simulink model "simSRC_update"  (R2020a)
settings: Solver=ode15s  StartTime=0.0  StopTime=tsim  FixedStep=tdelay/2  RelTol=1e-3
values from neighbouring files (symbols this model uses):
  d0 = 0    [runSRC.m]    (also in Main.m = [Fh, Tcin, Thin]; Main_OL.m = [Fh, Tcin, Thin]; runTestCalcBlk.m = [Fh, Tcin, Thin]; runTransf.m = [Fh, Tcin, Thin,U0])
  df = 0    [runSRC.m]
  h0 = x0    [runSRC.m]
  hf = h0    [runSRC.m]
  hmax = [2.3; 2.8; 3.2]    [runSRC.m]    (also in TuneSRC.m)
  nd = length(d0)    [runSRC.m]    (also in Main.m = size(d0,2); Main_OL.m = size(d0,2); runTestCalcBlk.m = size(d0,2); runTransf.m = size(d0,2))
  np = length(param)    [runSRC.m]    (also in runH2Psim.m; Main.m = size(p,2); Main_OL.m = size(p,2); runTestCalcBlk.m = size(p,2))
  nu = length(z0)    [runSRC.m]    (also in runH2Psim.m = length(u0); Main.m = 1; Main_OL.m = 1; runTestCalcBlk.m = 1)
  nx = length(x0)    [runSRC.m]    (also in H2P_Turbine_driven.m = param(end); runTD.m; H2P_Boiler_driven.m = param(end); runBD.m)
  param = [A; Cv; DP; rho; N]    [runSRC.m]    (also in TuneSRC.m = [vmin; vmax; umin; umax; n; price;opening]; runTD.m = [Tref;TrefB;dHvap;cpg;cpW;cpSt;R;Mwt;     T0;TG0;ME;pC;     ; runBD.m = [Tref;TrefB;dHvap;cpg;cpW;cpSt;R;Mwt;          T0;TG0;ME;pC;; runFP.m = [Tref;TrefB;dHvap;cpg;cpW;cpSt;R;Mwt;          T0;TG0;ME;pC;)
  pSR1 = [u01, alpha1, MV]    [runSRC.m]
  pSR2 = [u02, alpha2, MV]    [runSRC.m]
  pSR3 = [u03, alpha3, MV]    [runSRC.m]
  td = 0    [runSRC.m]
  tdelay = 1    [runSRC.m]
  th = ones(6,1)    [runSRC.m]
  v0 = v(end,:)    [runTD.m]    (also in runBD.m; runFP.m; runFPV2.m; runVPC.m)
  x0 = pr/100*hmax    [runSRC.m]    (also in TuneSRC.m = [hH; hH; hH].*hmax; runTD.m = [TE0;TD0;TSh0;MD0; MSh0;w0;TA0;0;0;0;0;0;0;0;0;0]; runBD.m = [TE0;TD0;TSh0;MD0; MSh0;w0;TA0;0;0;0;0;0;0;0;0;0]; runFP.m = [TE0;TD0;TSh0;MD0; MSh0;w0;TA0;0;0;0;0;0;0;0])
  z0 = [0.6; 0.7; 0.8; 1]    [runSRC.m]    (also in TuneSRC.m; runTD.m = [TGE0;TGD;TGSh;pT; Pm0;mG;zV]; runBD.m = [TGE0;TGD;TGSh;pT; Pm0;mG;zV]; runFP.m = [TGE0;TGD;TGSh;pT; Pm0;mG;zV])
  zOP = zOP0-[0.7;0;0;0]    [runSRC.m]
undefined symbols (not defined in the file or in its folder): KcSRC, KISRC, TanksODE, tzOP

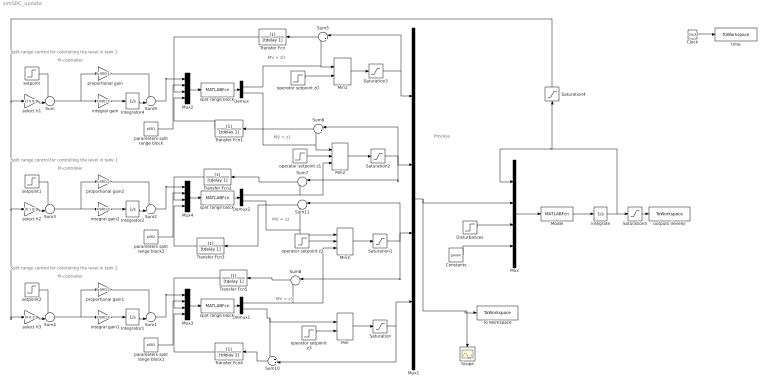
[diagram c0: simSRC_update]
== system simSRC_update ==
  note: MV = z3
  note: MV = z2
  note: MV = z1
  note: MV = z0
  note: Process
  note: Split range control for controlling the level in tank 1
  note: PI-controller
  note: PI-controller
  note: Split range control for controlling the level in tank 2
  note: PI-controller
  note: Split range control for controlling the level in tank 1
  Clock : Clock
  Constants : Constant  Value=param
  Demux : Demux  Outputs=2
  Demux1 : Demux  Outputs=2
  Demux2 : Demux  Outputs=2
  Disturbances : Step  Time=td  Before=d0  After=df  SampleTime=0
  Integrator1 : Integrator  InitialCondition=v0(3)
  Integrator2 : Integrator  InitialCondition=v0(2)
  Integrator4 : Integrator  InitialCondition=v0(1)
  Min : MinMax  Inputs=2
  Min1 : MinMax  Inputs=2
  Min2 : MinMax  Inputs=3
  Min3 : MinMax  Inputs=3
  Model : MATLABFcn  MATLABFcn=TanksODE(u(1:nx),u(nx+1:nx+nu),u(nx+nu+1:nx+nu+nd),u(nx+nu+nd+1:nx+nu+nd+np))  OutputDimensions=nx
  Mux{,1..4} (5 alike) : Mux
  Saturation{,1..3} (4 alike) : Saturate  UpperLimit=1  LowerLimit=0
  Saturation4 : Saturate  UpperLimit=hmax  LowerLimit=0
  Saturation5 : Saturate  UpperLimit=hmax  LowerLimit=0
  Scope : Scope
  Sum{,3..4,10} (4 alike) : Sum  Inputs=+-|
  Sum1 : Sum  Inputs=++|
  Sum{5..8,11} (5 alike) : Sum  Inputs=|-+
  Sum2 : Sum  Inputs=++|
  Sum9 : Sum  Inputs=++|
  To Workspace : ToWorkspace  VariableName=uSRC  SampleTime=-1
  Transfer Fcn{,1..5} (6 alike) : TransferFcn  Denominator=[tdelay 1]
  integral gain : Gain  Gain=KISRC(1)  Multiplication=Matrix(K*u)
  integral gain1 : Gain  Gain=KISRC(3)  Multiplication=Matrix(K*u)
  integral gain2 : Gain  Gain=KISRC(2)  Multiplication=Matrix(K*u)
  integrate : Integrator  InitialCondition=x0
  operator setpoint  z3 : Step  Time=tzOP(4)  Before=z0(4)  After=zOP(4)  SampleTime=0
  operator setpoint z0 : Step  Time=tzOP(1)  Before=z0(1)  After=zOP(1)  SampleTime=0
  operator setpoint z1 : Step  Time=tzOP(2)  Before=z0(2)  After=zOP(2)  SampleTime=0
  operator setpoint z2 : Step  Time=tzOP(3)  Before=z0(3)  After=zOP(3)  SampleTime=0
  outputs (levels) : ToWorkspace  VariableName=ySRC  SampleTime=-1
  parameters split range block : Constant  Value=pSR1
  parameters split range block1 : Constant  Value=pSR3
  parameters split range block2 : Constant  Value=pSR2
  proportional gain : Gain  Gain=KcSRC(1)  Multiplication=Matrix(K*u)
  proportional gain1 : Gain  Gain=KcSRC(3)  Multiplication=Matrix(K*u)
  proportional gain2 : Gain  Gain=KcSRC(2)  Multiplication=Matrix(K*u)
  select h1 : Gain  Gain=[1 0 0]  Multiplication=Matrix(K*u)
  select h2 : Gain  Gain=[0 1 0]  Multiplication=Matrix(K*u)
  select h3 : Gain  Gain=[0 0 1]  Multiplication=Matrix(K*u)
  setpoint : Step  Time=th(1)  Before=h0(1)  After=hf(1)  SampleTime=0
  setpoint1 : Step  Time=th(3)  Before=h0(2)  After=hf(2)  SampleTime=0
  setpoint2 : Step  Time=th(5)  Before=h0(3)  After=hf(3)  SampleTime=0
  "split range block " : MATLABFcn  MATLABFcn=SRblock_update(u(1),u(2:end-2),u(end-1:end))  OutputDimensions=2
  "split range block " : MATLABFcn  MATLABFcn=SRblock_update(u(1),u(2:end-2),u(end-1:end))  OutputDimensions=2
  "split range block " : MATLABFcn  MATLABFcn=SRblock_update(u(1),u(2:end-2),u(end-1:end))  OutputDimensions=2
  time : ToWorkspace  VariableName=tSRC  SampleTime=-1
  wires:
  Clock/1 -> time/1
  Mux/1 -> Model/1
  Model/1 -> integrate/1
  integrate/1 -> Saturation5/1, Mux/1, Saturation4/1
  Constants/1 -> Mux/4
  Disturbances/1 -> Mux/3
  Mux1/1 -> Scope/1, To Workspace/1, Mux/2
  Saturation3/1 -> Sum5/1, Mux1/1
  Saturation2/1 -> Sum7/1, Sum6/1, Mux1/2
  Saturation1/1 -> Sum11/1, Sum8/1, Mux1/3
  Saturation/1 -> Sum10/2, Mux1/4
  Min/1 -> Saturation/1
  Min2/1 -> Saturation2/1
  Min3/1 -> Saturation1/1
  Min1/1 -> Saturation3/1
  operator setpoint z0/1 -> Min1/2
  operator setpoint  z3/1 -> Min/2
  operator setpoint z2/1 -> Min3/2
  operator setpoint z1/1 -> Min2/2
  Sum/1 -> proportional gain/1, integral gain/1
  Integrator4/1 -> Sum9/2
  integral gain/1 -> Integrator4/1
  proportional gain/1 -> Sum9/1
  Sum9/1 -> Mux2/1
  Mux2/1 -> "split range block "/1
  parameters split range block/1 -> Mux2/2
  "split range block "/1 -> Demux/1
  Demux/1 -> Sum5/2, Min1/1
  Demux/2 -> Sum6/2, Min2/1
  Sum1/1 -> Mux3/1
  parameters split range block1/1 -> Mux3/2
  Mux3/1 -> "split range block "/1
  integral gain1/1 -> Integrator1/1
  Integrator1/1 -> Sum1/2
  Demux1/2 -> Sum10/1, Min/1
  "split range block "/1 -> Demux1/1
  Sum4/1 -> proportional gain1/1, integral gain1/1
  Demux1/1 -> Min3/3, Sum8/2
  proportional gain1/1 -> Sum1/1
  Sum2/1 -> Mux4/1
  parameters split range block2/1 -> Mux4/2
  Mux4/1 -> "split range block "/1
  integral gain2/1 -> Integrator2/1
  Integrator2/1 -> Sum2/2
  Demux2/2 -> Sum11/2, Min3/1
  "split range block "/1 -> Demux2/1
  Sum3/1 -> proportional gain2/1, integral gain2/1
  Demux2/1 -> Sum7/2, Min2/3
  proportional gain2/1 -> Sum2/1
  Saturation4/1 -> select h3/1, select h2/1, select h1/1
  select h1/1 -> Sum/2
  setpoint/1 -> Sum/1
  select h2/1 -> Sum3/2
  setpoint1/1 -> Sum3/1
  select h3/1 -> Sum4/2
  setpoint2/1 -> Sum4/1
  Transfer Fcn2/1 -> Mux4/3
  Saturation5/1 -> outputs (levels)/1
  Transfer Fcn/1 -> Mux2/3
  Transfer Fcn4/1 -> Mux3/4
  Transfer Fcn5/1 -> Mux3/3
  Transfer Fcn3/1 -> Mux4/4
  Transfer Fcn1/1 -> Mux2/4
  Sum5/1 -> Transfer Fcn/1
  Sum6/1 -> Transfer Fcn1/1
  Sum7/1 -> Transfer Fcn2/1
  Sum8/1 -> Transfer Fcn5/1
  Sum10/1 -> Transfer Fcn4/1
  Sum11/1 -> Transfer Fcn3/1
